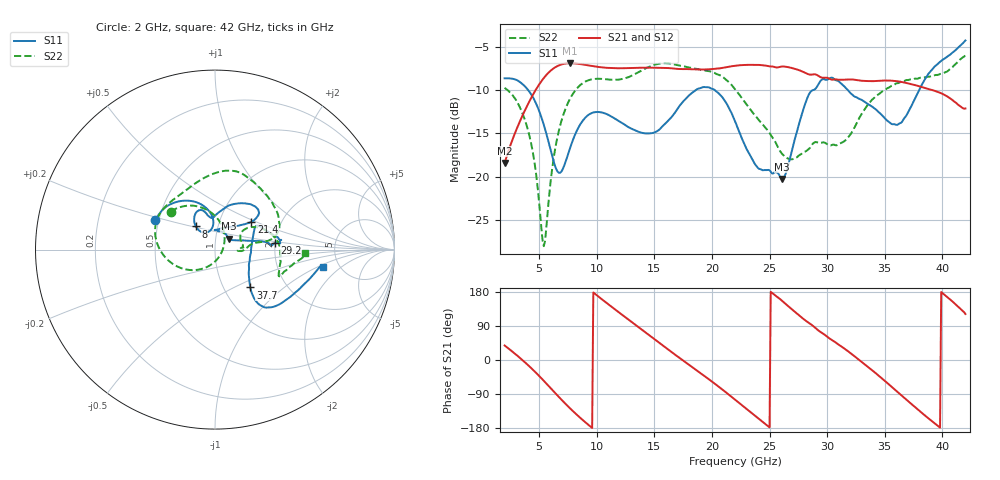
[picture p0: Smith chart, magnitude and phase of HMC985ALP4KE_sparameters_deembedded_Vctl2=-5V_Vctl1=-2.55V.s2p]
!s2p File: Measurements: S11, S21, S12, S22
# GHz S dB R 50.0
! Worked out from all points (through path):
!   401 points, 2 GHz to 42 GHz, reference 50 ohm
!   highest |S21| = -6.91 dB at 7.7 GHz (marker M1); lowest = -18.4 dB at 2 GHz (marker M2)
!   lowest |S11| = -20.3 dB at 26.1 GHz (marker M3), VSWR 1.22, Z = 57.7 + j7.07 ohm
!   |S11| at or under -10 dB: 4.039 GHz to 18.6 GHz (14.56 GHz wide, 129 % of centre); 20.23 GHz to 28.8 GHz (8.569 GHz wide, 35 % of centre); 31.79 GHz to 37.98 GHz (6.19 GHz wide, 17.7 % of centre)
!   |S22| runs from -28.0 to -6.0 dB; largest |S21 - S12| = 0.00044
!   S11 on the Smith chart (normalised r, x): 2 GHz: 0.48, +0.18; 8 GHz: 0.78, +0.21; 21.4 GHz: 1.41, +0.47; 29.2 GHz: 2.00, +0.17; 37.7 GHz: 1.33, -0.61; 42 GHz: 3.74, -1.18
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2  -8.65 153.9  -18.43 38.4  -18.44 38.4  -9.75 139.4
4  -9.93 121.1  -11.70 -12.5  -11.71 -12.5  -14.49 90.1
5.4  -14.01 96.4  -8.62 -54.8  -8.62 -54.8  -28.02 -24.4
6.7  -19.54 110.3  -7.17 -97.2  -7.17 -97.2  -14.75 -141.7
7.7  -16.63 130.2  -6.91 -128.2  -6.91 -128.2  -10.95 -172.2
8  -15.52 129.6  -6.92 -136.9  -6.92 -136.9  -10.29 -179.5
8.7  -13.70 124.3  -7.04 -156.2  -7.04 -156.2  -9.29 166.0
10.4  -12.58 110.2  -7.38 161.2  -7.39 161.3  -8.72 141.1
12.4  -13.97 102.7  -7.48 114.7  -7.49 114.7  -8.67 116.2
15.4  -14.60 90.6  -7.45 45.6  -7.46 45.6  -6.98 79.0
18.2  -10.40 58.8  -7.61 -16.5  -7.61 -16.5  -7.45 53.2
21.4  -11.89 37.5  -7.33 -89.9  -7.33 -89.9  -9.02 13.9
22  -13.57 41.7  -7.20 -104.6  -7.21 -104.6  -9.90 10.4
24.2  -19.12 87.2  -7.12 -158.3  -7.12 -158.3  -13.66 8.8
26.1  -20.25 38.6  -7.29 155.9  -7.29 155.9  -17.38 -3.3
28.7  -10.05 4.1  -8.21 91.7  -8.22 91.8  -16.28 4.7
29.2  -9.44 6.5  -8.33 78.9  -8.34 78.9  -16.08 4.6
32.5  -10.81 25.5  -8.84 6.8  -8.84 6.8  -13.99 34.2
35.4  -13.72 6.7  -8.91 -65.5  -8.91 -65.4  -9.69 14.7
37.7  -10.80 -47.1  -9.46 -126.2  -9.46 -126.2  -8.69 -6.0
39.7  -6.85 -44.7  -10.26 -176.0  -10.26 -175.9  -8.21 -22.6
42  -4.28 -9.3  -12.13 121.5  -12.14 121.5  -5.98 -2.1
